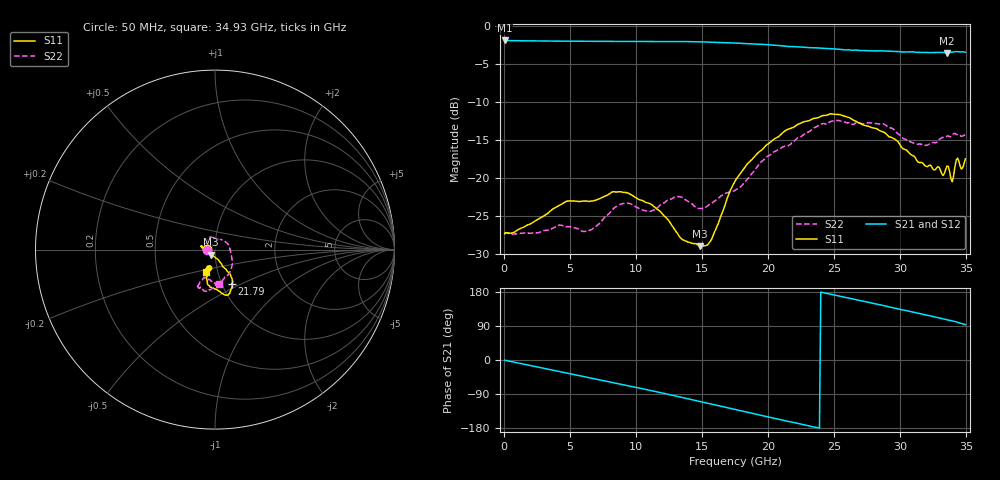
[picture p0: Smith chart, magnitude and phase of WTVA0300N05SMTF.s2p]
! 50 ohm 2-Port S-parameters measured by Modelithics Inc support@modelithics.com  Tampa, FL USA 813-866-6335 (February 2024)
! Smiths Interconnect,  3dB P/N: WTVA0300N05SMTF, Temperature: 125 C
! Board: 10 mil Rogers 4350B, Mounting Pad Dimensions: Length: 15 mils, Width: 25 mils, Gap: 40 mils.
# Hz S RI R 50
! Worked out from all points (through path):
!   352 points, 50 MHz to 34.93 GHz, reference 50 ohm
!   highest |S21| = -1.90 dB at 50 MHz (marker M1); lowest = -3.5 dB at 33.53 GHz (marker M2)
!   group delay of S21, straight-line fit = 21.2 ps
!   lowest |S11| = -29.0 dB at 14.83 GHz (marker M3), VSWR 1.07, Z = 47.8 - j2.69 ohm
!   |S11| at or under -10 dB: start of sweep to end of sweep
!   |S22| runs from -27.5 to -12.4 dB; largest |S21 - S12| = 0.0085
!   S11 on the Smith chart (normalised r, x): 50 MHz: 0.92, +0.00; 21.79 GHz: 1.12, -0.45; 34.93 GHz: 0.88, -0.22
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5e7  -0.0428 0.00146  0.8038 -0.00487  0.8028 -0.00461  -0.0424 0.000186
2.787e9  -0.053 0.0136  0.7487 -0.2749  0.7475 -0.2749  -0.044 0.00252
4.18e9  -0.0649 0.0104  0.6882 -0.399  0.6869 -0.3986  -0.048 -0.00902
5.8715e9  -0.0678 0.0172  0.5876 -0.5345  0.5868 -0.5338  -0.0433 -0.0104
8.8565e9  -0.0783 0.0201  0.3485 -0.7112  0.3463 -0.7108  -0.067 -0.00108
1.1742e10  -0.0609 0.00196  0.0639 -0.7876  0.0622 -0.7865  -0.0451 0.0468
1.30355e10  -0.0438 -0.00477  -0.0722 -0.7864  -0.0736 -0.7853  -0.0353 0.0668
1.48265e10  -0.0216 -0.0281  -0.26 -0.7428  -0.2612 -0.741  0.0125 0.0616
1.5722e10  -0.00401 -0.0393  -0.3478 -0.7009  -0.3481 -0.6992  0.0451 0.0506
1.7513e10  0.0394 -0.0872  -0.502 -0.5881  -0.5017 -0.5867  0.0826 0.00567
1.98015e10  0.0848 -0.1385  -0.6453 -0.3932  -0.6445 -0.3923  0.093 -0.0983
2.17915e10  0.0952 -0.1915  -0.7042 -0.2028  -0.7034 -0.2014  0.0496 -0.1629
2.33835e10  0.0874 -0.2291  -0.7181 -0.0502  -0.7171 -0.0503  -0.00905 -0.2105
2.5473e10  0.057 -0.2538  -0.686 0.149  -0.6849 0.1489  -0.0637 -0.2277
2.91545e10  -0.0418 -0.1812  -0.5255 0.4376  -0.5203 0.4413  -0.0896 -0.194
3.19405e10  -0.0377 -0.113  -0.3229 0.5867  -0.3206 0.5865  -0.0481 -0.1559
3.3234e10  -0.0318 -0.0984  -0.2124 0.6358  -0.2084 0.636  -0.0147 -0.1841
3.35325e10  -0.0352 -0.1142  -0.1862 0.6389  -0.1813 0.639  -0.00946 -0.1877
3.39305e10  -0.0289 -0.0895  -0.153 0.6553  -0.148 0.6552  0.00651 -0.19
3.4229e10  -0.0493 -0.1208  -0.1234 0.6674  -0.118 0.667  0.00484 -0.1934
3.4627e10  -0.0356 -0.1084  -0.0726 0.6722  -0.0725 0.6706  0.00842 -0.1874
3.49255e10  -0.0514 -0.123  -0.0414 0.6716  -0.0408 0.67  0.0199 -0.1916
